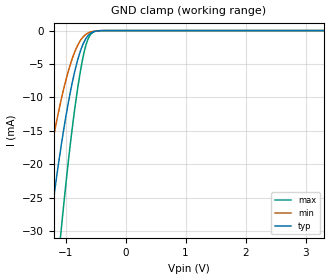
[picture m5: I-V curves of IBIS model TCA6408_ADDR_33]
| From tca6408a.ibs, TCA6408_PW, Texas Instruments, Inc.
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[Model]   TCA6408_ADDR_33
Model_type  Input
Vinl=0.9
Vinh=2.52
| variable   typ   min   max
C_comp   2.21pF   1.76pF   2.42pF
[Temperature Range]   40   100   -40
| Ambient temperature   25   85   -40
[Voltage range]   3.3   3   3.6
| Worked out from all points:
|   GND clamp passes 1 mA (typ) near -0.65 V on its own axis
[GND Clamp]
| TCA6408_ADDR_33
|   Voltage   I(typ)   I(min)   I(max)
-3.3V     -229.8mA   -173.1mA   -314.8mA
-1.49V    -47mA      -31.57mA   -73.96mA
-1.455V   -44.17mA   -29.5mA    -69.9mA
-1.285V   -31.19mA   -20.13mA   -51.01mA
-1.255V   -29.05mA   -18.6mA    -47.84mA
-1.08V    -17.66mA   -10.65mA   -30.52mA
-945mV    -10.37mA   -5.81mA    -18.9mA
-810mV    -4.799mA   -2.428mA   -9.366mA
-700mV    -1.861mA   -882.4uA   -3.61mA
-615mV    -655uA     -320.4uA   -1.07mA
-410mV    -13.36uA   -10.66uA   -11.01uA
3.3V      289.3pA    1.025nA    57.78pA
